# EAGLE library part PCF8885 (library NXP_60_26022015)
NXP Capacitive 8-channel proximity switch with auto-calibration and very low power consumption AAL Eindhoven MK
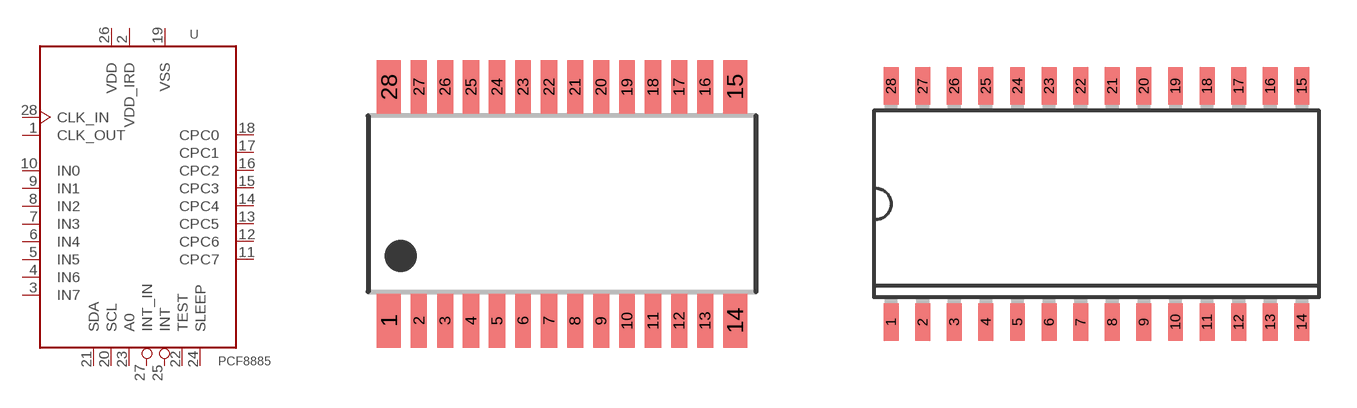
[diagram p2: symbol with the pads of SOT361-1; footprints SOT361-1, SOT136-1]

Designator prefix U

## PCF8885TS  [SOT361-1]
1  CLK_OUT  out
2  VDD_IRD  pwr
3  IN7  in
4  IN6  in
5  IN5  in
6  IN4  in
7  IN3  in
8  IN2  in
9  IN1  in
10  IN0  in
11  CPC7  pas
12  CPC6  pas
13  CPC5  pas
14  CPC4  pas
15  CPC3  pas
16  CPC2  pas
17  CPC1  pas
18  CPC0  pas
19  VSS  pwr
20  SCL  in
21  SDA
22  TEST  in
23  A0  in
24  SLEEP  in
25  INT  out
26  VDD  pwr
27  INT_IN  in
28  CLK_IN  in

## PCF8885T  [SOT136-1]
Pads as for SOT361-1

## Footprint SOT361-1 (pad centres in mm)
SOT361-1 TSSOP28: plastic thin shrink small outline package; 28 leads; body width 4.4 mm JEDEC: MO-153 IEC: ---
smd 0.6 x 1.35: 1 -4.325,-2.925; 14 4.325,-2.925; 15 4.325,2.925; 28 -4.325,2.925
smd 0.4 x 1.35: 2 -3.575,-2.925; 3 -2.925,-2.925; 4 -2.275,-2.925; 5 -1.625,-2.925; 6 -0.975,-2.925; 7 -0.325,-2.925; 8 0.325,-2.925; 9 0.975,-2.925; 10 1.625,-2.925; 11 2.275,-2.925; 12 2.925,-2.925; 13 3.575,-2.925; 16 3.575,2.925; 17 2.925,2.925; 18 2.275,2.925; 19 1.625,2.925; 20 0.975,2.925; 21 0.325,2.925; 22 -0.325,2.925; 23 -0.975,2.925; 24 -1.625,2.925; 25 -2.275,2.925; 26 -2.925,2.925; 27 -3.575,2.925

## Footprint SOT136-1 (pad centres in mm)
SOT136-1 SO28: plastic small outline package; 28 leads; body width 7.5 mm JEDEC: MS-013 IEC: 075E06
smd 0.6 x 1.5: 1 -8.255,-4.75; 2 -6.985,-4.75; 3 -5.715,-4.75; 4 -4.445,-4.75; 5 -3.175,-4.75; 6 -1.905,-4.75; 7 -0.635,-4.75; 8 0.635,-4.75; 9 1.905,-4.75; 10 3.175,-4.75; 11 4.445,-4.75; 12 5.715,-4.75; 13 6.985,-4.75; 14 8.255,-4.75; 15 8.255,4.75; 16 6.985,4.75; 17 5.715,4.75; 18 4.445,4.75; 19 3.175,4.75; 20 1.905,4.75; 21 0.635,4.75; 22 -0.635,4.75; 23 -1.905,4.75; 24 -3.175,4.75; 25 -4.445,4.75; 26 -5.715,4.75; 27 -6.985,4.75; 28 -8.255,4.75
